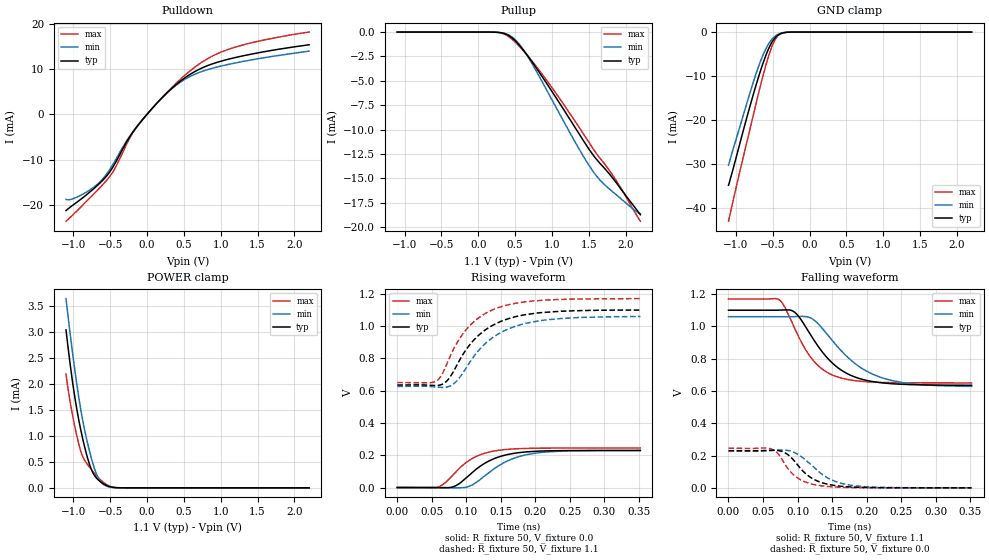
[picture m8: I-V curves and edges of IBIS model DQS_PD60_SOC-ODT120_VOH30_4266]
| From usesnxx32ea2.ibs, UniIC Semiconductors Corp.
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| DQS_PD60_SOC-ODT120_VOH30_4266
| (60 Ohm Pulldown, 120 Ohm System ODT Setting, VOH=VDDQ/3.0, 3200-4266Mbps)
[Model]   DQS_PD60_SOC-ODT120_VOH30_4266
Model_type   I/O
Vinl = 123.333mV
Vinh = 243.333mV
Vmeas = 183.333mV
Vref = 0.0mV
Cref = 0.0pF
Rref = 120.000Ohm
|   typ   min   max
|C_comp   0.849pF   0.799pF   0.899pF
C_comp_pullup   0.4245pF   0.3995pF   0.4495pF
C_comp_pulldown   0.4245pF   0.3995pF   0.4495pF
| Note: C_comp changes when the ODT circuit is enabled.
[Model Spec]
| Input threshold voltage corners
Vinl   0.1233V   0.1167V   0.1350V
Vinh   0.2433V   0.2367V   0.2550V
| Measurement voltage corners
Vmeas   0.1833V   0.1767V   0.1950V
| Timing spec test load voltage corners
Vref   0.0000V   0.0000V   0.0000V
| Dynamic Overshoot Parameters from LPDDR4 Specification
D_overshoot_ampl_h   0.30   NA   NA
D_overshoot_ampl_l   0.30   NA   NA
D_overshoot_area_h   0.1n   NA   NA
D_overshoot_area_l   0.1n   NA   NA
[Voltage Range]   1.1000V   1.0600V   1.1700V
[Pullup Reference]   1.1000V   1.0600V   1.1700V
| Junction Temperature (Ambient temp is 35C typ 95C min -40C max)
[Temperature Range]   50.0   110.0   -40.0
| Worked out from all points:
|   slope of the pulldown table from 0 to 0.165 V, typ, clamps not added: 55 ohm
|   slope of the pullup table from 0 to 0.165 V, typ, clamps not added: 39.2 kohm
|   GND clamp passes 1 mA (typ) near -0.45 V on its own axis
|   POWER clamp passes 1 mA (typ) near -0.88 V on its own axis
|   rising waveform, R_fixture 50, V_fixture 0.0: 20-80 % time 47.1ps typ, 51.2ps min, 41.8ps max; typ from 0 V to 0.23 V
|   falling waveform, R_fixture 50, V_fixture 1.1: 20-80 % time 53.3ps typ, 65ps min, 42.9ps max; typ from 1.1 V to 0.635 V
|   rising waveform, R_fixture 50, V_fixture 1.1: 20-80 % time 56.3ps typ, 60.3ps min, 52.3ps max; typ from 0.635 V to 1.1 V
|   falling waveform, R_fixture 50, V_fixture 0.0: 20-80 % time 35ps typ, 42.4ps min, 30.4ps max; typ from 0.23 V to 0 V
[Pulldown]
|   Voltage   I(typ)   I(min)   I(max)
-1.1V     -21.25mA   -18.78mA   -23.61mA
-918.5mV  -19mA      -18.02mA   -20.81mA
-638mV    -15.16mA   -14.89mA   -16.16mA
-453.2mV  -11.38mA   -10.78mA   -12.45mA
-235.4mV  -4.998mA   -4.872mA   -5.302mA
-116.6mV  -2.307mA   -2.303mA   -2.296mA
276.1mV   4.816mA    4.74mA     4.918mA
437.8mV   7.121mA    6.906mA    7.497mA
625.9mV   9.213mA    8.675mA    10.1mA
880mV     11.08mA    10.12mA    12.78mA
1.144V    12.31mA    11.14mA    14.54mA
2.2V      15.34mA    13.95mA    18.15mA
[GND Clamp]
|   Voltage   I(typ)   I(min)   I(max)
-1.1V     -34.74mA   -30.21mA   -42.91mA
-948.2mV  -25.43mA   -21.63mA   -31.79mA
-793.1mV  -15.92mA   -12.96mA   -20.95mA
-723.8mV  -11.93mA   -9.348mA   -16.1mA
-664.4mV  -8.736mA   -6.578mA   -12.07mA
-591.8mV  -5.254mA   -3.789mA   -7.492mA
-525.8mV  -2.766mA   -1.974mA   -3.964mA
-469.7mV  -1.356mA   -986uA     -1.787mA
-416.9mV  -597.3uA   -440.2uA   -665.1uA
-357.5mV  -190.9uA   -145.2uA   -173.7uA
-265.1mV  -19.48uA   -16.92uA   -12.31uA
2.2V      0A         0A         0A
[Pullup]
|   Voltage   I(typ)   I(min)   I(max)
-1.1V     2.092uA    3.224uA    943.2nA
233.2mV   -16.12uA   -16.27uA   -16.87uA
335.5mV   -114uA     -94.77uA   -157uA
441.1mV   -501.8uA   -411.9uA   -628.2uA
556.6mV   -1.342mA   -1.243mA   -1.448mA
678.7mV   -2.516mA   -2.582mA   -2.496mA
1.055V    -6.719mA   -7.703mA   -6.276mA
1.362V    -10.35mA   -11.89mA   -9.685mA
1.553V    -12.54mA   -14.22mA   -11.89mA
1.675V    -13.64mA   -15.35mA   -13.14mA
1.867V    -15.37mA   -16.63mA   -15.15mA
2.2V      -18.72mA   -18.61mA   -19.39mA
[POWER Clamp]
|   Voltage   I(typ)   I(min)   I(max)
-1.1V     3.033mA    3.633mA    2.184mA
-1.041V   2.345mA    2.929mA    1.625mA
-984.5mV  1.782mA    2.31mA     1.205mA
-911.9mV  1.201mA    1.61mA     764.1uA
-852.5mV  818.2uA    1.148mA    543.5uA
-776.6mV  434.1uA    683.3uA    390.2uA
-710.6mV  232.2uA    359uA      273.1uA
-657.8mV  146.8uA    178.8uA    190.6uA
-595.1mV  80.78uA    68.3uA     109.2uA
-482.9mV  15.69uA    9.499uA    19.51uA
-364.1mV  1.098uA    819.7nA    867nA
2.2V      0A         0A         0A
[Ramp]
|   typ   min   max
| 20% - 80%
dV/dt_r   137.76m/47.06p   137.31m/51.22p   146.97m/41.83p
dV/dt_f   278.79m/53.28p   259.05m/65.05p   312.06m/42.98p
| 25% - 75%
|dV/dt_r   114.80m/37.54p   114.43m/40.90p   122.47m/33.22p
|dV/dt_f   232.32m/42.47p   215.88m/51.80p   260.05m/34.24p
R_load = 50
[Rising Waveform]
R_fixture = 50
V_fixture = 0.0
|   Time   V(typ)   V(min)   V(max)
0s        225.3uV    184.2uV    168.8uV
58ps      -235.5uV   253.1uV    2.338mV
68ps      -877.8uV   -528.5uV   24.86mV
80ps      3.421mV    -1.491mV   74.85mV
107ps     87.78mV    12.87mV    175.8mV
124ps     143.1mV    62.63mV    208.8mV
143ps     183.7mV    124.3mV    228.2mV
170ps     212.5mV    182.9mV    239.5mV
205ps     225.5mV    215.6mV    243.8mV
352ps     229.8mV    229mV      245.1mV
[Falling Waveform]
R_fixture   = 50
V_fixture   = 1.1
V_fixture_min = 1.06
V_fixture_max = 1.17
|   Time   V(typ)   V(min)   V(max)
0s        1.1V       1.06V      1.17V
75ps      1.101V     1.06V      1.16V
96ps      1.087V     1.06V      986.5mV
119ps     947mV      1.052V     809.1mV
135ps     846.2mV    992.1mV    738mV
157ps     748.6mV    878.7mV    687.9mV
190ps     676.5mV    748.8mV    660.6mV
227ps     648.3mV    675.4mV    652.5mV
272ps     638.4mV    641.6mV    650.3mV
352ps     635.4mV    628.2mV    649.9mV
[Rising Waveform]
R_fixture   = 50
V_fixture   = 1.1
V_fixture_min = 1.06
V_fixture_max = 1.17
|   Time   V(typ)   V(min)   V(max)
0s        635mV      626.1mV    649.8mV
58ps      632.2mV    621.6mV    664.1mV
65ps      639.4mV    619.9mV    702.1mV
74ps      670.3mV    624.7mV    787.4mV
86ps      755.2mV    659.1mV    892.9mV
99ps      849.6mV    735.8mV    973.7mV
121ps     954.6mV    864mV      1.06V
146ps     1.021V     950.2mV    1.114V
211ps     1.084V     1.036V     1.16V
352ps     1.099V     1.059V     1.17V
[Falling Waveform]
R_fixture = 50
V_fixture = 0.0
|   Time   V(typ)   V(min)   V(max)
0s        229.9mV    229.2mV    245.2mV
59ps      232.6mV    229.9mV    244.5mV
69ps      232.8mV    232.8mV    222.5mV
77ps      226.2mV    234.3mV    179.5mV
98ps      152.9mV    213.6mV    67.75mV
113ps     83.32mV    168mV      33.78mV
130ps     40.1mV     102.6mV    15.5mV
154ps     14.49mV    40.75mV    5.262mV
186ps     3.913mV    11.43mV    1.37mV
352ps     303.3uV    314.6uV    191.7uV
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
